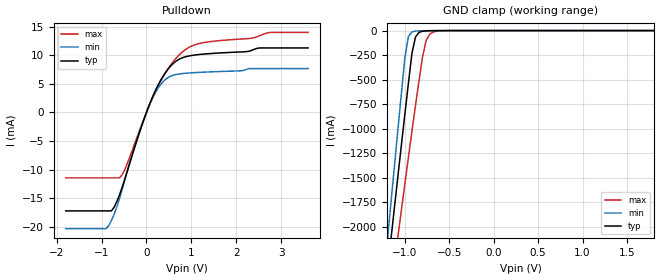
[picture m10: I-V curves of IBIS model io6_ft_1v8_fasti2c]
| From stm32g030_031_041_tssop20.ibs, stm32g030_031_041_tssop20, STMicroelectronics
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[Model]  io6_ft_1v8_fasti2c
Model_type I/O_open_drain
Polarity   Non-Inverting
Enable   Active-Low
Vinl =   0.540000V
Vinh =   1.260000V
Vmeas =  0.90000V
Cref =   30.000000pF
Rref =   500
Vref =   3.0V
C_comp   1.277600pF   1.236700pF   1.315100pF
[Temperature Range]   25.000000   -40.000000   0.125000k
[Pullup Reference]   1.800000V   1.600000V   2.000000V
[Pulldown Reference]   0.0V   0.0V   0.0V
[POWER Clamp Reference]   1.800000V   1.600000V   2.000000V
[GND Clamp Reference]   0.0V   0.0V   0.0V
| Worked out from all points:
|   slope of the pulldown table from 0 to 0.27 V, typ, clamps not added: 54.7 ohm
|   GND clamp passes 1 mA (typ) near -0.66 V on its own axis
[Pulldown]
|Voltage   I(typ)   I(min)   I(max)
-1.8V     -17.22mA   -20.33mA   -11.45mA
-900mV    -17.22mA   -20.33mA   -11.45mA
-720mV    -16.58mA   -17.82mA   -11.45mA
-600mV    -14.41mA   -15.08mA   -11.45mA
-480mV    -11.58mA   -11.79mA   -9.954mA
0V        10fA       11fA       0A
240mV     4.49mA     3.999mA    4.291mA
480mV     7.563mA    6.085mA    7.612mA
780mV     9.487mA    6.76mA     10.43mA
1.14V     10.08mA    6.976mA    11.96mA
2.76V     11.26mA    7.652mA    13.98mA
3.6V      11.26mA    7.652mA    13.98mA
[GND_clamp]
|Voltage   I(typ)   I(min)   I(max)
-1.8V     -7.471A    -7.973A    -7.298A
-1.2V     -2.489A    -2.18A     -2.954A
-1.16V    -2.16A     -1.797A    -2.674A
-1.08V    -1.505A    -1.034A    -2.118A
-1V       -857.9mA   -283.1mA   -1.568A
-960mV    -540.4mA   -62.14mA   -1.296A
-920mV    -234.4mA   -13.75mA   -1.028A
-880mV    -66.29mA   -4.855mA   -765.3mA
-800mV    -6.505mA   -2.056mA   -266mA
-760mV    -3.074mA   -1.45mA    -100.4mA
-680mV    -1.215mA   -557.1uA   -14.19mA
1.8V      0A         0A         0A
[POWER_clamp]
|Voltage   I(typ)   I(min)   I(max)
-1.8V     0A         0A         0A
0V        0A         0A         0A
[Ramp]
| variable   typ   min   max
dV/dt_r  0.306/4.06140n   0.211/4.37750n   0.370/4.25525n
dV/dt_f  0.30570/3.93750n   0.21030/4.44000n   0.37008/3.81562n
R_load = 50.000000
